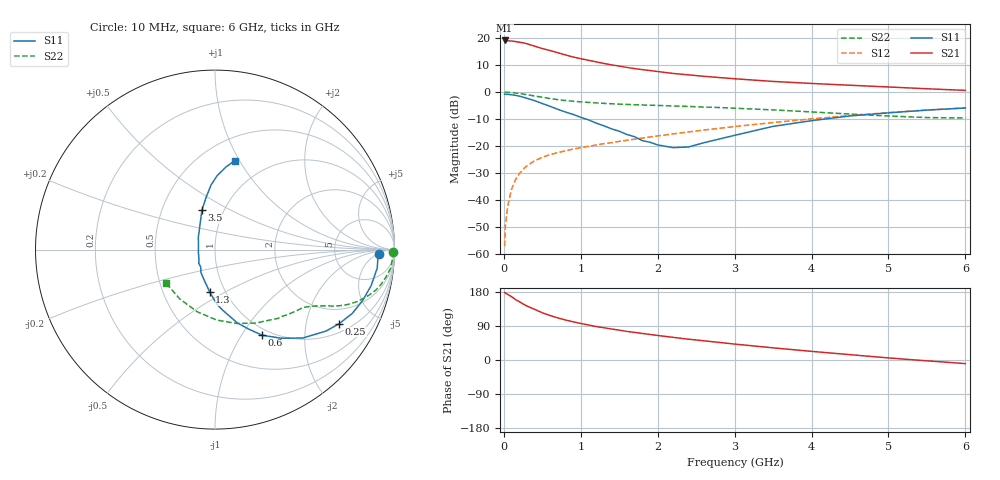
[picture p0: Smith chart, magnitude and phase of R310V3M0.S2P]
! SIEMENS Small Signal Semiconductors
! BFR181
! Si NPN RF Bipolar Junction Transistor in SOT23
! VCE = 10 V  IC = 3 mA
! Common Emitter S-Parameters:  May  1996
# GHz  S  MA  R  50
!  f  S11  S21  S12  S22
! GHz  MAG  ANG  MAG  ANG  MAG  ANG  MAG  ANG
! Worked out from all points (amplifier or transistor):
!   36 points, 10 MHz to 6 GHz, reference 50 ohm
!   highest |S21| = 19.1 dB at 10 MHz (marker M1)
!   |S21| within 3 dB of that: start of sweep to 500.1 MHz
!   unconditionally stable (mu >= 1): 1.467 GHz to 3.335 GHz
!   at 250 MHz: K = 0.30, MSG = 23.4 dB, |S12| = -28.6 dB
!   at 1.4 GHz: K = 0.99, MSG = 14.4 dB, |S12| = -18.7 dB
!   at 6 GHz: K = 0.86, MSG = 3.2 dB, |S12| = -5.8 dB
!   S11 on the Smith chart (normalised r, x): 10 MHz: 21, -6; 250 MHz: 1.32, -3.11; 600 MHz: 0.91, -1.24; 1.3 GHz: 0.85, -0.42; 3.5 GHz: 0.79, +0.37; 6 GHz: 0.72, +0.96
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0.01  0.9145 -1.4  9.049 178.1  0.0014 96.0  0.9943 -0.7
0.02  0.9088 -2.6  9.002 176.7  0.0033 79.9  0.9917 -1.4
0.05  0.9098 -6.5  8.898 173.2  0.0077 84.8  0.99 -3.2
0.1  0.8927 -13.0  8.833 167.1  0.0158 82.9  0.9832 -6.2
0.15  0.871 -18.8  8.641 159.8  0.0236 78.0  0.9637 -9.3
0.25  0.8058 -30.8  8.191 147.9  0.0373 72.5  0.9222 -14.3
0.3  0.7671 -36.3  7.857 142.4  0.043 70.5  0.8949 -16.5
0.4  0.6941 -45.2  7.1 133.7  0.0535 66.1  0.8468 -19.9
0.5  0.6147 -53.4  6.407 124.6  0.0618 63.4  0.8016 -22.4
0.6  0.5453 -61.1  5.886 117.4  0.0694 61.2  0.7605 -24.3
0.7  0.4813 -67.0  5.375 111.2  0.0756 60.0  0.7256 -25.7
0.8  0.4274 -73.0  4.883 105.6  0.0816 58.9  0.6976 -26.7
0.9  0.3866 -76.9  4.471 100.8  0.0881 58.5  0.6777 -27.6
1.1  0.3061 -87.8  3.886 92.4  0.0991 58.3  0.6438 -29.2
1.3  0.2376 -97.2  3.395 85.1  0.1109 58.5  0.6183 -30.6
1.6  0.164 -115.1  2.863 75.4  0.1281 59.0  0.591 -33.0
2.2  0.0936 -171.2  2.217 59.8  0.1682 58.8  0.5537 -39.5
3  0.1582 122.2  1.767 42.0  0.23 56.0  0.5026 -50.9
3.5  0.2319 108.3  1.576 32.1  0.2731 52.8  0.4683 -60.9
4.5  0.3616 93.4  1.34 14.1  0.3681 43.9  0.3925 -88.7
5.5  0.464 82.5  1.153 -2.2  0.4654 32.1  0.3376 -125.5
6  0.5077 77.4  1.076 -9.5  0.5108 25.2  0.3312 -146.2
